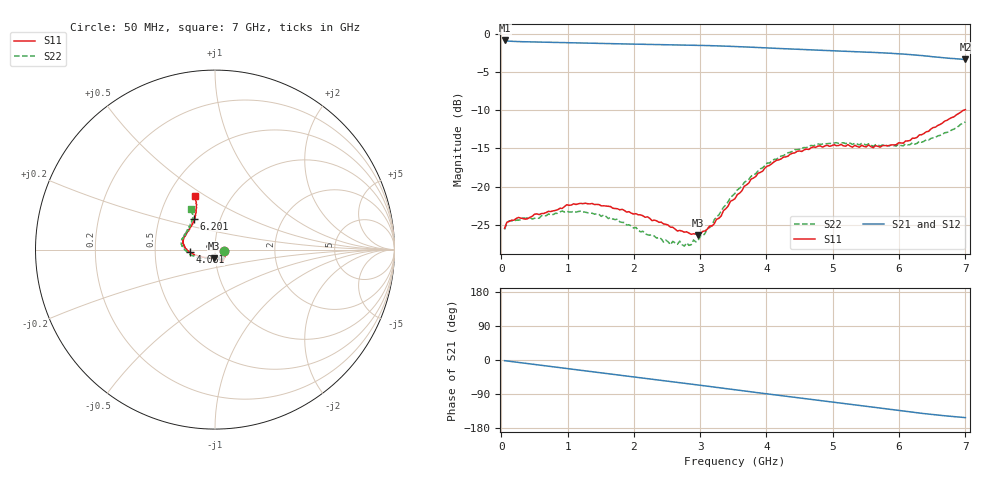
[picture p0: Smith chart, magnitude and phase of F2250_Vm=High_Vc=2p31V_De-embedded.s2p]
! Integrated Device Technology
! Corporate Headquarters
! 6024 Silver Creek Valley Road
! San Jose, CA 95138  USA
! Phone:  1-408-284-8200
! Toll Free:  1-800-223-1366
! Webpage:  http://www.idt.com/
! Timing and RF Division
! 515 Groton Road, Suite 102
! Westford, MA 01886-6024
! Device:  F2250
! Description: Voltage Variable RF Attenuator
! Frequency:  50.0 -  6000.00 MHz
! Package:  3x3 mm Thin QFN Plastic Package: 16 pin
! Ports:  2 RF, 3 DC
!  Pin  1  = GND
!  Pin  2  = NC
!  Pin  3  = RF1  = Port 1
!  Pin  4  = NC
!  Pin  5  = GND
!  Pin  6  = GND
!  Pin  7  = GND
!  Pin  8  = GND
!  Pin  9  = NC
!  Pin 10  = RF2  = Port 2
!  Pin 11  = NC
!  Pin 12  = GND
!  Pin 13  = GND
!  Pin 14  = VCNTRL
!  Pin 15  = VDD
!  Pin 16  = VMODE
! Vcntrl:  2.310 Volts
! Vmode:  +3.300 Volts
! Vdd:  +3.30  Volts
! Current:  1.315 mA
! Data:  The device was measured on a the F2250 evaluation board which has
!  individual transmission lines to the RF pins.  Data was collected
!  using a calibrated network analyzer.  The evaluation board was
!  de-embedded using a TRL calibration technique.
!  The reference plane is the edge of the package pin.
! Misc:  SN 10
!  Action Tracker AT0258
! Date Measured:  2014-11-26
! Date:  2015-10-15  MJV
! Note:
!  Integrated Device Technology supplies this data as a sample of measured
!  data at the package pin for this product.  Your particular data for this
!  product may vary.
!  Data was taken at 25 degrees C.
!  Integrated Device Technology reserves the right to change this data at anytime.
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# GHz S dB R 50
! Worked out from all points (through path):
!   201 points, 50 MHz to 7 GHz, reference 50 ohm
!   highest |S21| = -0.91 dB at 50 MHz (marker M1); lowest = -3.4 dB at 7 GHz (marker M2)
!   group delay of S21, straight-line fit = 61.2 ps
!   lowest |S11| = -26.3 dB at 2.969 GHz (marker M3), VSWR 1.10, Z = 49.2 - j4.75 ohm
!   |S11| at or under -10 dB: start of sweep to 6.98 GHz
!   |S22| runs from -27.8 to -11.5 dB; largest |S21 - S12| = 0.0019
!   S11 on the Smith chart (normalised r, x): 50 MHz: 1.11, -0.02; 4.081 GHz: 0.75, -0.02; 6.201 GHz: 0.75, +0.27; 7 GHz: 0.68, +0.45
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0.05  -25.42 -10.4  -0.91 -1.8  -0.90 -1.8  -25.59 -10.7
0.1195  -24.52 -10.0  -1.00 -3.2  -1.00 -3.2  -24.47 -8.8
0.57125  -23.63 -30.8  -1.12 -13.3  -1.12 -13.3  -24.12 -31.1
0.91875  -22.84 -49.4  -1.19 -21.0  -1.19 -21.1  -23.17 -50.6
1.2315  -22.21 -57.1  -1.25 -27.9  -1.25 -27.9  -23.30 -61.1
1.75275  -22.87 -64.1  -1.34 -39.1  -1.34 -39.1  -24.22 -67.6
2.37825  -24.65 -63.9  -1.44 -52.8  -1.44 -52.8  -26.61 -67.2
2.552  -25.28 -68.7  -1.46 -56.7  -1.46 -56.7  -27.57 -73.6
2.691  -25.70 -76.5  -1.49 -59.8  -1.49 -59.8  -27.10 -81.2
2.7605  -25.94 -78.7  -1.50 -61.3  -1.50 -61.3  -27.76 -85.6
2.969  -26.31 -96.4  -1.54 -66.0  -1.54 -66.0  -27.02 -104.9
3.1775  -25.13 -119.3  -1.59 -70.7  -1.59 -70.7  -25.05 -126.4
3.525  -21.56 -151.7  -1.69 -78.5  -1.69 -78.6  -20.87 -148.5
3.76825  -19.00 -164.0  -1.79 -84.0  -1.79 -84.0  -18.63 -159.5
4.081  -16.99 -175.1  -1.91 -91.0  -1.91 -91.0  -16.67 -171.3
4.4285  -15.57 176.4  -2.04 -98.6  -2.05 -98.6  -15.16 178.8
4.7065  -14.80 169.5  -2.14 -104.8  -2.15 -104.8  -14.65 173.1
5.054  -14.64 161.3  -2.27 -112.5  -2.27 -112.5  -14.25 166.0
5.85325  -14.61 135.4  -2.57 -130.0  -2.57 -130.1  -14.66 147.3
6.20075  -13.66 123.8  -2.78 -137.7  -2.78 -137.8  -14.24 138.3
6.54825  -12.23 115.8  -3.05 -144.7  -3.05 -144.9  -13.58 126.9
7  -9.94 110.9  -3.38 -152.1  -3.39 -152.2  -11.54 120.7
